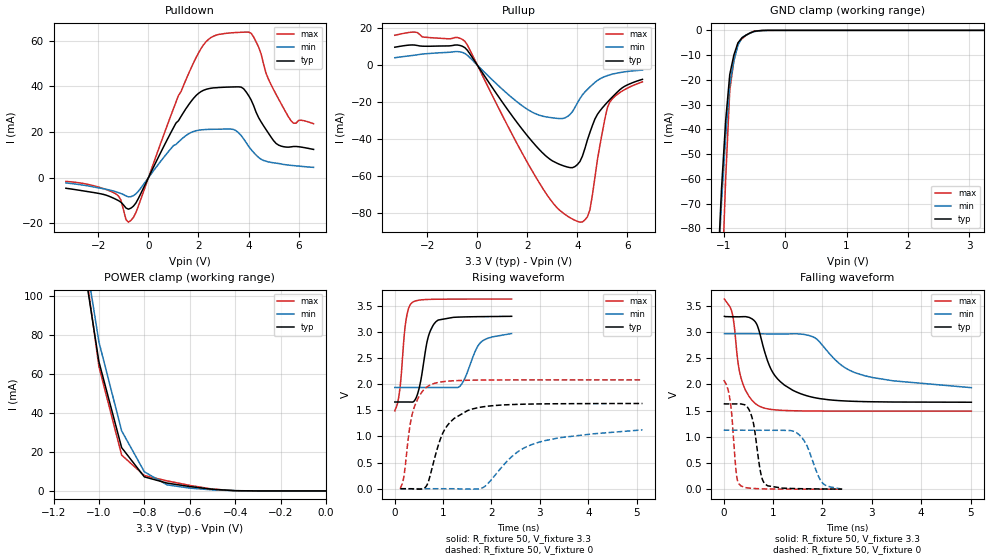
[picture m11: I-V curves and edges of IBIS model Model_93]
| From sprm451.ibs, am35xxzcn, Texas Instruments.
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| Model based on original model for BQ1833DV50BTPBFZP18LL_7LM_X50
|   Sub model LM_X50_PD_PU_OFF_3P3
[model]   Model_93
|[Description]  3.3V-I/O-PI-X
|[Input Load]   PI
|[Output Drive]
|Voltage   3.3V
|Mode   I/O
Model_type   I/O
Polarity   Non-Inverting
Enable   Active-Low
Vinl =  0.8V
Vinh =  2V
Cref =  15pF
Rref =  100.0000M
Vref =  0V
Vmeas =  1.65
C_comp   1.683006p   1.492615p   1.787227p
[Model Spec]
Vinl   0.8V   0.8V   0.8V
Vinh   2V   2V   2V
[Temperature Range]   25   125   -40
[Voltage Range]   3.3   2.97   3.63
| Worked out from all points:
|   slope of the pulldown table from 0 to 0.495 V, typ, clamps not added: 44.5 ohm
|   slope of the pullup table from 0 to 0.495 V, typ, clamps not added: 49.1 ohm
|   GND clamp passes 1 mA (typ) near -0.56 V on its own axis
|   POWER clamp passes 1 mA (typ) near -0.51 V on its own axis
|   rising waveform, R_fixture 50, V_fixture 3.3: 20-80 % time 195ps typ, 279ps min, 122ps max; typ from 1.66 V to 3.3 V
|   rising waveform, R_fixture 50, V_fixture 0: 20-80 % time 428ps typ, 982ps min, 236ps max; typ from 0 V to 1.63 V
|   falling waveform, R_fixture 50, V_fixture 3.3: 20-80 % time 497ps typ, 969ps min, 226ps max; typ from 3.3 V to 1.66 V
|   falling waveform, R_fixture 50, V_fixture 0: 20-80 % time 155ps typ, 285ps min, 110ps max; typ from 1.63 V to 0 V
[POWER_clamp]
-3.3V     2.414A     2.856A     2.597A
-1.067V   116.4mA    125.1mA    120.2mA
-1.033V   91.29mA    100.7mA    91.93mA
-1V       66.19mA    76.32mA    63.69mA
-900mV    22.2mA     30.8mA     18.38mA
-800mV    7.208mA    9.795mA    7.881mA
-700mV    4.017mA    3.114mA    5.155mA
-600mV    2.246mA    1.437mA    2.828mA
-500mV    840.1uA    538.7uA    942.1uA
-400mV    133.3uA    110.7uA    103.8uA
0V        9.333nA    42.82nA    36.63nA
[Pulldown]
-3.3V     -4.669mA   -2.345mA   -1.683mA
-1.3V     -9.527mA   -6.237mA   -7.18mA
-900mV    -13.33mA   -8.043mA   -18.4mA
-700mV    -13.38mA   -8.364mA   -18.74mA
1.8V      34.72mA    20.23mA    50.28mA
2.3V      38.67mA    21.09mA    59.54mA
2.8V      39.47mA    21.22mA    62.74mA
3.5V      39.76mA    20.55mA    63.58mA
4.1V      34.11mA    12.32mA    63.3mA
5V        16.21mA    6.486mA    38.59mA
5.7V      13.47mA    5.354mA    24.85mA
6.6V      12.34mA    4.484mA    23.64mA
[Pullup]
-3.3V     9.738mA    4.045mA    16.21mA
-2.5V     10.91mA    5.432mA    17.94mA
-500mV    9.5mA      6.347mA    12.96mA
1.4V      -27.68mA   -17.82mA   -37.78mA
2.4V      -44.64mA   -26.76mA   -62.11mA
3.5V      -54.84mA   -28.6mA    -80.92mA
4.1V      -52.27mA   -18.13mA   -85.16mA
4.5V      -36.47mA   -11.82mA   -78.33mA
5V        -23.1mA    -6.724mA   -36.03mA
5.2V      -20.04mA   -5.652mA   -22.93mA
5.3V      -18.59mA   -5.203mA   -19.89mA
6.6V      -7.68mA    -2.683mA   -9.05mA
[GND_clamp]
-3.3V     -1.975A    -1.766A    -3.378A
-1.1V     -99.4mA    -100.8mA   -162mA
-1.033V   -63.74mA   -69.32mA   -106.1mA
-966.7mV  -36.56mA   -43.04mA   -60.17mA
-900mV    -17.88mA   -22mA      -24.31mA
-833.3mV  -9.995mA   -12.37mA   -12.32mA
-766.7mV  -5.035mA   -6.016mA   -5.345mA
-700mV    -2.995mA   -2.928mA   -3.372mA
-566.7mV  -1.037mA   -1.089mA   -982.7uA
-500mV    -379.4uA   -508.9uA   -286.6uA
-300mV    -14.25uA   -22.31uA   -14.38uA
3.233V    8.935nA    10.41uA    33.57nA
[Ramp]
dV/dt_f  0.9840264/0.49685831n 0.61917332/0.96340423n  1.2838169/0.22527997n
dV/dt_r  0.9837651/0.42618919n 0.68058631/0.97768791n  1.2549258/0.23334898n
R_load = 50
[Rising Waveform]
R_fixture = 50
V_fixture = 3.3
V_fixture_min = 2.97
V_fixture_max = 3.63
4.379ps   1.66V      1.938V     1.49V
103.5ps   1.66V      1.938V     1.87V
241ps     1.66V      1.938V     3.254V
360.3ps   1.658V     1.938V     3.562V
502.4ps   1.907V     1.938V     3.609V
703.9ps   2.934V     1.938V     3.623V
855.1ps   3.198V     1.938V     3.627V
1.331ns   3.285V     1.948V     3.629V
1.774ns   3.294V     2.796V     3.63V
2.416ns   3.3V       2.97V      3.63V
[Rising Waveform]
R_fixture = 50
V_fixture = 0
V_fixture_min = 0
V_fixture_max = 0
119.2ps   8.36nV     112.1nV    4.117nV
189.8ps   2.491uV    -318.3nV   223mV
380.5ps   -2.93mV    -54.86nV   1.486V
623.8ps   17.23mV    189.9nV    1.913V
736.3ps   259.3mV    75.4nV     1.986V
1.027ns   1.122V     8.582uV    2.052V
1.506ns   1.495V     -7.118mV   2.076V
1.856ns   1.572V     39.84mV    2.081V
2.835ns   1.621V     845.6mV    2.083V
5.119ns   1.631V     1.126V     2.083V
[Falling Waveform]
R_fixture = 50
V_fixture = 3.3
V_fixture_min = 2.97
V_fixture_max = 3.63
15.01ps   3.3V       2.97V      3.63V
175.2ps   3.292V     2.97V      3.346V
295.7ps   3.291V     2.97V      2.38V
385.8ps   3.294V     2.97V      2.015V
611.3ps   3.225V     2.969V     1.66V
737.4ps   2.952V     2.966V     1.578V
1.03ns    2.177V     2.964V     1.515V
1.612ns   1.804V     2.956V     1.494V
2.837ns   1.672V     2.17V      1.49V
5.015ns   1.66V      1.938V     1.49V
[Falling Waveform]
R_fixture = 50
V_fixture = 0
V_fixture_min = 0
V_fixture_max = 0
0s        1.631V     1.126V     2.083V
127.2ps   1.628V     1.126V     1.708V
259.7ps   1.628V     1.126V     272.1mV
347.3ps   1.628V     1.126V     63.24mV
570.1ps   1.379V     1.125V     15.44mV
746.7ps   322.6mV    1.124V     7.312mV
834.1ps   101.5mV    1.124V     4.71mV
1.523ns   9.731mV    1.044V     154.9uV
1.979ns   3.941mV    143.3mV    21.24uV
2.4ns     8.36nV     112.1nV    4.117nV
